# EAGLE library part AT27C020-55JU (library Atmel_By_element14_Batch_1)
2-Megabit OTP EPROM
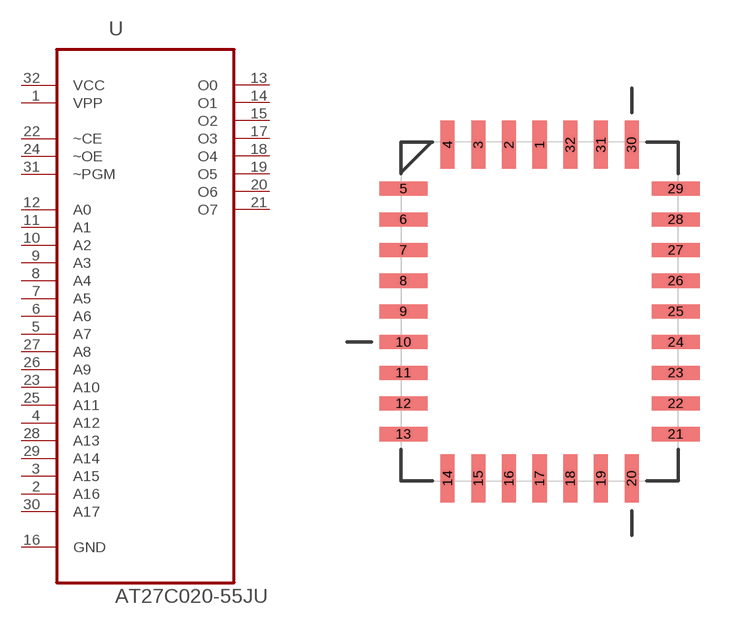
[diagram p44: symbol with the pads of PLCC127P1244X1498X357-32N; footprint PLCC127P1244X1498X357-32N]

Designator prefix U

## AT27C020-55JU (DESCRIPTION: 2-Megabit OTP EPROM; MPN: AT27C020-55JU; OC_FARNELL: 1455020; OC_NEWARK: 58M3819; PACKAGE: PLCC-32; SUPPLIER: Atmel Corporation)  [PLCC127P1244X1498X357-32N]
1  VPP  pwr
2  A16  in
3  A15  in
4  A12  in
5  A7  in
6  A6  in
7  A5  in
8  A4  in
9  A3  in
10  A2  in
11  A1  in
12  A0  in
13  O0  out
14  O1  out
15  O2  out
16  GND  pas
17  O3  out
18  O4  out
19  O5  out
20  O6  out
21  O7  out
22  ~CE  in
23  A10  in
24  ~OE  in
25  A11  in
26  A9  in
27  A8  in
28  A13  in
29  A14  in
30  A17  in
31  ~PGM  in
32  VCC  pwr

## Footprint PLCC127P1244X1498X357-32N (pad centres in mm)
smd 0.584 x 1.981: 1 0,6.909; 2 -1.27,6.909; 3 -2.54,6.909; 4 -3.81,6.909; 14 -3.81,-6.909; 15 -2.54,-6.909; 16 -1.27,-6.909; 17 0,-6.909; 18 1.27,-6.909; 19 2.54,-6.909; 20 3.81,-6.909; 30 3.81,6.909; 31 2.54,6.909; 32 1.27,6.909
smd 1.981 x 0.584: 5 -5.639,5.08; 6 -5.639,3.81; 7 -5.639,2.54; 8 -5.639,1.27; 9 -5.639,0; 10 -5.639,-1.27; 11 -5.639,-2.54; 12 -5.639,-3.81; 13 -5.639,-5.08; 21 5.639,-5.08; 22 5.639,-3.81; 23 5.639,-2.54; 24 5.639,-1.27; 25 5.639,0; 26 5.639,1.27; 27 5.639,2.54; 28 5.639,3.81; 29 5.639,5.08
